| TEXAS INSTRUMENTS INCORPORATED
| Standard Linear and Logic Group
| IBIS Model of SN74AVCH20T245
| 20-BIT DUAL-SUPPLY BUS TRANSCEIVER WITH CONFIGURABLE VOLTAGE
| TRANSLATION AND 3-STATE OUTPUTS
| This file contains package information for the following:
|  TVSOP 56-pin (DGV) package as [Component] AVCH20T245_DGV
|  VFBGA 56-pin (GQL) package as [Component] AVCH20T245_GQL
|  TSSOP 56-pin (DGG) package as [Component] AVCH20T245_DGG
| This device can be powered at the following Vccs:
|  1.2 volt Vcc
|  1.5 volt Vcc
|  1.8 volt Vcc
|  2.5 volt Vcc
|  3.3 volt Vcc
| This file provides unique models under the [Model Selector] for each Vcc.
| For operation at a specific Vcc, select the appropriate model after each
| [Model Selector] keyword.
[IBIS Ver]   3.2
[Comment char]  |_char
[File Name]   sn74avch20t245.ibs
[File Rev]   1.2 | x_die
[Date]   April 20, 2004
[Source]   Data created from TI-SPICE simulations at TI-SLL.
[Notes]   The following is an IBIS list for the AVCH20T245.
   Please contact sllibis@ti.com with questions and
   comments concerning SLL IBIS models.
   - FILE REV HISTORY
   - 1.2 Release of GQL package on 04/20/04
   - Power clamp data deleted as there is no power-clamp diode.
   - Due to the fact that the Device is 4.6-V Input/Output
   tolarent, the I/O models has some Non-Monotonic Warnings.
   - Non-monotonic data in ground-clamp due to bus-hold
[Disclaimer] Property of Texas Instruments Incorporated.  Unauthorized
   reproduction and/or distribution is strictly prohibited.
   This product is protected under copyright law.
   Created  2003, (C) Copyright  2003, Texas Instruments
   Incorporated, All Rights Reserved
   UNLESS THERE IS A SIGNED, WRITTEN AGREEMENT TO THE
   CONTRARY, TEXAS INSTRUMENTS (TI) IS PROVIDING THE IBIS
   MODELS  AND WITHOUT ANY WARRANTY, EXPRESSED OR
   IMPLIED.  TI assumes no liability for:
   1) the accuracy of the IBIS models provided to your
   company;
   2) the proper functioning of these IBIS Models in your
   design or for any resulting applications; or
   3) infringement of patents, copyrights or intellectual
   property rights resulting from your use of these IBIS
   models.
   TI provides IBIS Models as a service to our customers.
   You and your company shall not distribute, sell or give
   these models to anyone else without prior written
   permission from TI.
   TI reserves the right to make changes to our products or
   to discontinue any semiconductor product or service
   without notice, and advises our customers to obtain the
   latest version of relevant information to verify, before
   placing orders, that the information being relied on is
   current.
   Please be aware that your receipt and use of the IBIS
   information provided shall serve as acceptance of these
   terms and conditions.  If you do not accept these terms,
   you should return or destroy the IBIS models and any
   other accompanying information immediately.
| Component AVCH20T245_DGV 56-pin TVSOP
[Component]   AVCH20T245_DGV
[Manufacturer]   Texas Instruments, Inc.
[Package]
|   typ   min   max
R_pkg   6.300e-02   5.000e-02   8.400e-02
L_pkg   2.945e-09   2.394e-09   3.939e-09
C_pkg   3.910e-13   2.710e-13   5.880e-13
[Pin]   signal_name   model_name   R_pin   L_pin   C_pin
1   1DIR   AVCH20T245_DIR   6.800e-02   3.933e-09   5.880e-13
2   1B1   AVCH20T245_IO   6.800e-02   3.568e-09   5.870e-13
3   1B2   AVCH20T245_IO   7.600e-02   3.464e-09   5.150e-13
4   GND   GND   8.400e-02   3.444e-09   4.590e-13
5   1B3   AVCH20T245_IO   8.100e-02   3.277e-09   4.270e-13
6   1B4   AVCH20T245_IO   7.400e-02   3.136e-09   3.870e-13
7   VCCB   POWER   6.900e-02   2.970e-09   4.010e-13
8   1B5   AVCH20T245_IO   5.000e-02   2.785e-09   3.790e-13
9   1B6   AVCH20T245_IO   5.100e-02   2.685e-09   3.200e-13
10   1B7   AVCH20T245_IO   5.300e-02   2.611e-09   3.160e-13
11   GND   GND   5.300e-02   2.495e-09   2.970e-13
12   1B8   AVCH20T245_IO   5.300e-02   2.435e-09   2.920e-13
13   1B9   AVCH20T245_IO   5.500e-02   2.412e-09   2.850e-13
14   1B10   AVCH20T245_IO   5.600e-02   2.401e-09   2.730e-13
15   2B1   AVCH20T245_IO   5.500e-02   2.401e-09   2.730e-13
16   2B2   AVCH20T245_IO   5.500e-02   2.399e-09   2.840e-13
17   2B3   AVCH20T245_IO   5.400e-02   2.406e-09   2.890e-13
18   GND   GND   5.300e-02   2.450e-09   2.930e-13
19   2B4   AVCH20T245_IO   5.100e-02   2.544e-09   3.110e-13
20   2B5   AVCH20T245_IO   5.100e-02   2.626e-09   3.150e-13
21   2B6   AVCH20T245_IO   5.000e-02   2.727e-09   3.690e-13
22   VCCB   POWER   6.500e-02   2.903e-09   3.930e-13
23   2B7   AVCH20T245_IO   7.500e-02   3.091e-09   3.860e-13
24   2B8   AVCH20T245_IO   8.200e-02   3.272e-09   4.280e-13
25   GND   GND   8.200e-02   3.393e-09   4.570e-13
26   2B9   AVCH20T245_IO   7.300e-02   3.380e-09   5.080e-13
27   2B10   AVCH20T245_IO   7.100e-02   3.577e-09   5.800e-13
28   2DIR   AVCH20T245_DIR   6.800e-02   3.937e-09   5.740e-13
29   2NOE   AVCH20T245_NOE   6.900e-02   3.923e-09   5.690e-13
30   2A10   AVCH20T245_IO   6.400e-02   3.536e-09   5.740e-13
31   2A9   AVCH20T245_IO   7.600e-02   3.428e-09   5.170e-13
32   GND   GND   8.100e-02   3.395e-09   4.680e-13
33   2A8   AVCH20T245_IO   8.000e-02   3.255e-09   4.310e-13
34   2A7   AVCH20T245_IO   7.100e-02   3.064e-09   3.860e-13
35   VCCA   POWER   6.100e-02   2.878e-09   3.890e-13
36   2A6   AVCH20T245_IO   5.000e-02   2.710e-09   3.630e-13
37   2A5   AVCH20T245_IO   5.000e-02   2.606e-09   3.110e-13
38   2A4   AVCH20T245_IO   5.200e-02   2.534e-09   3.060e-13
39   GND   GND   5.200e-02   2.439e-09   2.890e-13
40   2A3   AVCH20T245_IO   5.300e-02   2.399e-09   2.860e-13
41   2A2   AVCH20T245_IO   5.500e-02   2.394e-09   2.820e-13
42   2A1   AVCH20T245_IO   5.500e-02   2.398e-09   2.710e-13
43   1A10   AVCH20T245_IO   5.600e-02   2.396e-09   2.710e-13
44   1A9   AVCH20T245_IO   5.400e-02   2.402e-09   2.830e-13
45   1A8   AVCH20T245_IO   5.400e-02   2.423e-09   2.880e-13
46   GND   GND   5.300e-02   2.474e-09   2.920e-13
47   1A7   AVCH20T245_IO   5.100e-02   2.569e-09   3.090e-13
48   1A6   AVCH20T245_IO   5.100e-02   2.638e-09   3.130e-13
49   1A5   AVCH20T245_IO   5.100e-02   2.742e-09   3.660e-13
50   VCCA   POWER   6.400e-02   2.917e-09   3.900e-13
51   1A4   AVCH20T245_IO   7.400e-02   3.083e-09   3.830e-13
52   1A3   AVCH20T245_IO   8.100e-02   3.249e-09   4.300e-13
53   GND   GND   8.300e-02   3.400e-09   4.550e-13
54   1A2   AVCH20T245_IO   7.500e-02   3.427e-09   5.050e-13
55   1A1   AVCH20T245_IO   7.100e-02   3.585e-09   5.780e-13
56   1NOE   AVCH20T245_NOE   6.900e-02   3.939e-09   5.810e-13
| Component AVCH20T245_GQL 56-pin jrBGA
[Component]   AVCH20T245_GQL
[Manufacturer]   Texas Instruments, Inc.
[Package]
|   typ   min   max
R_pkg   6.500e-02   3.500e-02   9.700e-02
L_pkg   1.952e-09   1.000e-09   3.191e-09
C_pkg   2.830e-13   1.620e-13   4.340e-13
[Pin]   signal_name   model_name   R_pin   L_pin   C_pin
 A3   1DIR   AVCH20T245_DIR   3.600e-02   1.004e-09   1.760e-13
 A2   1B2   AVCH20T245_IO   4.000e-02   1.191e-09   1.860e-13
 A1   1B1   AVCH20T245_IO   4.700e-02   1.411e-09   2.090e-13
 B3   GND   GND   9.700e-02   3.191e-09   4.340e-13
 B2   1B4   AVCH20T245_IO   7.400e-02   2.213e-09   3.290e-13
 B1   1B3   AVCH20T245_IO   6.000e-02   1.712e-09   2.430e-13
 C3   VCCB   POWER   8.500e-02   2.691e-09   3.680e-13
 C2   1B6   AVCH20T245_IO   7.400e-02   2.160e-09   3.150e-13
 C1   1B5   AVCH20T245_IO   6.000e-02   1.666e-09   2.470e-13
 D2   1B8   AVCH20T245_IO   7.400e-02   2.121e-09   3.130e-13
 D3   GND   GND   9.100e-02   2.924e-09   3.970e-13
 D1   1B7   AVCH20T245_IO   6.000e-02   1.619e-09   2.450e-13
 E2   1B10   AVCH20T245_IO   6.900e-02   2.031e-09   2.880e-13
 E1   1B9   AVCH20T245_IO   6.000e-02   1.583e-09   2.200e-13
 F1   2B1   AVCH20T245_IO   6.000e-02   1.578e-09   2.200e-13
 F2   2B2   AVCH20T245_IO   6.900e-02   2.017e-09   2.860e-13
 G1   2B3   AVCH20T245_IO   6.000e-02   1.594e-09   2.410e-13
 G3   GND   GND   9.200e-02   2.917e-09   3.970e-13
 G2   2B4   AVCH20T245_IO   7.500e-02   2.114e-09   3.150e-13
 H1   2B5   AVCH20T245_IO   6.000e-02   1.632e-09   2.470e-13
 H2   2B6   AVCH20T245_IO   7.000e-02   2.074e-09   3.070e-13
 H3   VCCB   POWER   8.600e-02   2.664e-09   3.650e-13
 J1   2B7   AVCH20T245_IO   6.000e-02   1.689e-09   2.490e-13
 J2   2B8   AVCH20T245_IO   6.600e-02   2.152e-09   3.320e-13
 J3   GND   GND   8.700e-02   3.118e-09   4.230e-13
 K1   2B9   AVCH20T245_IO   3.800e-02   1.303e-09   2.000e-13
 K2   2B10   AVCH20T245_IO   3.500e-02   1.176e-09   1.830e-13
 K3   2DIR   AVCH20T245_DIR   3.500e-02   1.007e-09   1.620e-13
 K4   2NOE   AVCH20T245_NOE   3.500e-02   1.000e-09   1.620e-13
 K5   2A10   AVCH20T245_IO   3.500e-02   1.154e-09   1.800e-13
 K6   2A9   AVCH20T245_IO   4.100e-02   1.352e-09   2.040e-13
 J4   GND   GND   8.800e-02   3.137e-09   4.300e-13
 J5   2A8   AVCH20T245_IO   7.400e-02   2.218e-09   3.340e-13
 J6   2A7   AVCH20T245_IO   6.000e-02   1.683e-09   2.500e-13
 H4   VCCA   POWER   8.500e-02   2.658e-09   3.720e-13
 H5   2A6   AVCH20T245_IO   7.500e-02   2.149e-09   3.210e-13
 H6   2A5   AVCH20T245_IO   6.000e-02   1.627e-09   2.480e-13
 G5   2A4   AVCH20T245_IO   7.500e-02   2.113e-09   3.140e-13
 G4   GND   GND   9.200e-02   2.922e-09   3.960e-13
 G6   2A3   AVCH20T245_IO   6.000e-02   1.594e-09   2.420e-13
 F5   2A2   AVCH20T245_IO   6.900e-02   2.016e-09   2.880e-13
 F6   2A1   AVCH20T245_IO   6.000e-02   1.580e-09   2.210e-13
 E6   1A9   AVCH20T245_IO   6.000e-02   1.582e-09   2.200e-13
 E5   1A10   AVCH20T245_IO   6.900e-02   2.026e-09   2.890e-13
 D6   1A7   AVCH20T245_IO   6.000e-02   1.610e-09   2.450e-13
 D4   GND   GND   9.200e-02   2.933e-09   3.960e-13
 D5   1A8   AVCH20T245_IO   7.500e-02   2.126e-09   3.110e-13
 C6   1A5   AVCH20T245_IO   6.000e-02   1.641e-09   2.450e-13
 C5   1A6   AVCH20T245_IO   7.300e-02   2.168e-09   3.190e-13
 C4   VCCA   POWER   8.600e-02   2.675e-09   3.620e-13
 B6   1A3   AVCH20T245_IO   6.000e-02   1.688e-09   2.430e-13
 B5   1A4   AVCH20T245_IO   7.500e-02   2.281e-09   3.330e-13
 B4   GND   GND   9.500e-02   3.168e-09   4.240e-13
 A6   1A1   AVCH20T245_IO   4.500e-02   1.418e-09   2.090e-13
 A5   1A2   AVCH20T245_IO   3.900e-02   1.216e-09   1.900e-13
 A4   1NOE   AVCH20T245_NOE   3.700e-02   1.029e-09   1.790e-13
| Component AVCH20T245_DGG 56-pin TSSOP
[Component]   AVCH20T245_DGG
[Manufacturer]   Texas Instruments, Inc.
[Package]
|   typ   min   max
R_pkg   4.500e-02   3.500e-02   6.200e-02
L_pkg   3.324e-09   2.403e-09   5.094e-09
C_pkg   5.640e-13   3.410e-13   9.140e-13
[Pin]   signal_name   model_name   R_pin   L_pin   C_pin
1   1DIR   AVCH20T245_DIR   6.200e-02   5.094e-09   8.560e-13
2   1B1   AVCH20T245_IO   6.100e-02   4.621e-09   9.020e-13
3   1B2   AVCH20T245_IO   6.000e-02   4.316e-09   8.020e-13
4   GND   GND   5.900e-02   3.968e-09   6.980e-13
5   1B3   AVCH20T245_IO   5.700e-02   3.716e-09   6.490e-13
6   1B4   AVCH20T245_IO   4.200e-02   3.517e-09   6.530e-13
7   VCCB   POWER   4.100e-02   3.160e-09   5.700e-13
8   1B5   AVCH20T245_IO   3.900e-02   2.981e-09   4.820e-13
9   1B6   AVCH20T245_IO   3.900e-02   2.808e-09   4.470e-13
10   1B7   AVCH20T245_IO   3.800e-02   2.715e-09   4.090e-13
11   GND   GND   4.100e-02   2.675e-09   3.910e-13
12   1B8   AVCH20T245_IO   3.900e-02   2.536e-09   3.660e-13
13   1B9   AVCH20T245_IO   3.900e-02   2.457e-09   3.480e-13
14   1B10   AVCH20T245_IO   3.800e-02   2.411e-09   3.530e-13
15   2B1   AVCH20T245_IO   3.900e-02   2.456e-09   3.550e-13
16   2B2   AVCH20T245_IO   3.900e-02   2.471e-09   3.490e-13
17   2B3   AVCH20T245_IO   4.000e-02   2.580e-09   3.700e-13
18   GND   GND   3.800e-02   2.651e-09   3.890e-13
19   2B4   AVCH20T245_IO   3.800e-02   2.739e-09   4.110e-13
20   2B5   AVCH20T245_IO   3.900e-02   2.838e-09   4.490e-13
21   2B6   AVCH20T245_IO   3.800e-02   2.988e-09   4.840e-13
22   VCCB   POWER   3.800e-02   3.104e-09   5.640e-13
23   2B7   AVCH20T245_IO   4.000e-02   3.427e-09   6.380e-13
24   2B8   AVCH20T245_IO   5.600e-02   3.654e-09   6.410e-13
25   GND   GND   5.700e-02   3.932e-09   7.000e-13
26   2B9   AVCH20T245_IO   5.800e-02   4.257e-09   8.060e-13
27   2B10   AVCH20T245_IO   5.700e-02   4.580e-09   9.140e-13
28   2DIR   AVCH20T245_DIR   5.900e-02   5.038e-09   8.610e-13
29   2NOE   AVCH20T245_NOE   6.000e-02   5.058e-09   8.580e-13
30   2A10   AVCH20T245_IO   5.600e-02   4.543e-09   9.040e-13
31   2A9   AVCH20T245_IO   5.700e-02   4.241e-09   8.020e-13
32   GND   GND   5.900e-02   3.933e-09   6.990e-13
33   2A8   AVCH20T245_IO   5.600e-02   3.616e-09   6.370e-13
34   2A7   AVCH20T245_IO   3.700e-02   3.368e-09   6.400e-13
35   VCCA   POWER   3.600e-02   3.024e-09   5.630e-13
36   2A6   AVCH20T245_IO   3.500e-02   2.876e-09   4.740e-13
37   2A5   AVCH20T245_IO   3.500e-02   2.745e-09   4.440e-13
38   2A4   AVCH20T245_IO   3.700e-02   2.683e-09   4.050e-13
39   GND   GND   3.800e-02   2.603e-09   3.820e-13
40   2A3   AVCH20T245_IO   3.800e-02   2.510e-09   3.620e-13
41   2A2   AVCH20T245_IO   3.600e-02   2.412e-09   3.410e-13
42   2A1   AVCH20T245_IO   3.800e-02   2.416e-09   3.490e-13
43   1A10   AVCH20T245_IO   3.800e-02   2.403e-09   3.490e-13
44   1A9   AVCH20T245_IO   3.700e-02   2.429e-09   3.410e-13
45   1A8   AVCH20T245_IO   3.600e-02   2.483e-09   3.580e-13
46   GND   GND   3.700e-02   2.614e-09   3.810e-13
47   1A7   AVCH20T245_IO   3.500e-02   2.669e-09   4.020e-13
48   1A6   AVCH20T245_IO   3.600e-02   2.763e-09   4.420e-13
49   1A5   AVCH20T245_IO   3.600e-02   2.942e-09   4.780e-13
50   VCCA   POWER   3.500e-02   3.053e-09   5.640e-13
51   1A4   AVCH20T245_IO   3.600e-02   3.408e-09   6.410e-13
52   1A3   AVCH20T245_IO   5.800e-02   3.698e-09   6.410e-13
53   GND   GND   5.900e-02   3.974e-09   6.970e-13
54   1A2   AVCH20T245_IO   6.100e-02   4.327e-09   8.020e-13
55   1A1   AVCH20T245_IO   6.100e-02   4.624e-09   9.050e-13
56   1NOE   AVCH20T245_NOE   6.000e-02   5.063e-09   8.580e-13
| Model AVCH20T245_NOE
[Model Selector]   AVCH20T245_NOE
AVCH20T245_NOE_12   1.2 volt Vcc
AVCH20T245_NOE_15   1.5 volt Vcc
AVCH20T245_NOE_18   1.8 volt Vcc
AVCH20T245_NOE_25   2.5 volt Vcc
AVCH20T245_NOE_33   3.3 volt Vcc
| Model AVCH20T245_DIR
[Model Selector]   AVCH20T245_DIR
AVCH20T245_DIR_12   1.2 volt Vcc
AVCH20T245_DIR_15   1.5 volt Vcc
AVCH20T245_DIR_18   1.8 volt Vcc
AVCH20T245_DIR_25   2.5 volt Vcc
AVCH20T245_DIR_33   3.3 volt Vcc
| Model AVCH20T245_IO
[Model Selector]   AVCH20T245_IO
AVCH20T245_IO_12   1.2 volt Vcc
AVCH20T245_IO_15   1.5 volt Vcc
AVCH20T245_IO_18   1.8 volt Vcc
AVCH20T245_IO_25   2.5 volt Vcc
AVCH20T245_IO_33   3.3 volt Vcc
| Models and submodels in the file (15): AVCH20T245_NOE_12 (Input), AVCH20T245_NOE_15 (Input), AVCH20T245_NOE_18 (Input), AVCH20T245_NOE_25 (Input), AVCH20T245_NOE_33 (Input), AVCH20T245_DIR_12 (Input), AVCH20T245_DIR_15 (Input), AVCH20T245_DIR_18 (Input), AVCH20T245_DIR_25 (Input), AVCH20T245_DIR_33 (Input), AVCH20T245_IO_12 (I/O), AVCH20T245_IO_15 (I/O), AVCH20T245_IO_18 (I/O), AVCH20T245_IO_25 (I/O), AVCH20T245_IO_33 (I/O)
